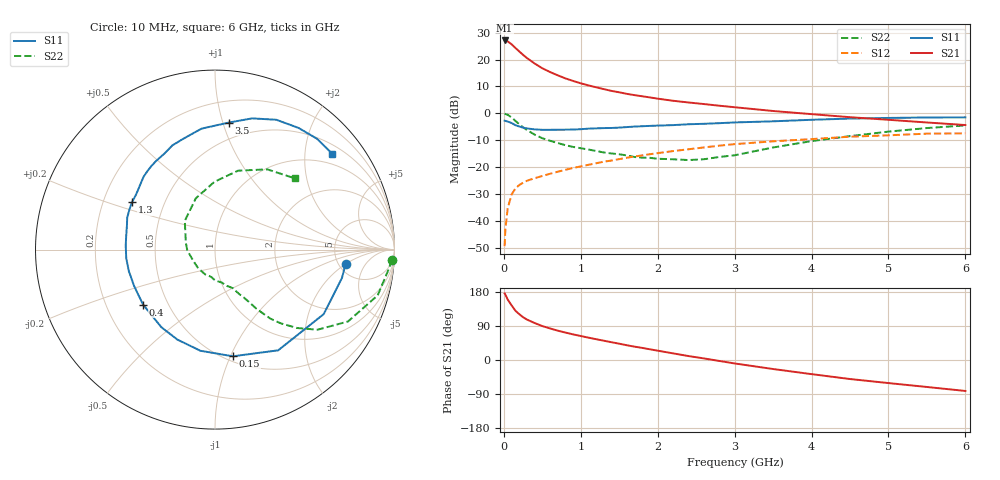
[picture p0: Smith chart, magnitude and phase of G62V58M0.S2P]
! SIEMENS Small Signal Semiconductors
! BFG193
! Si NPN RF Bipolar Junction Transistor in SOT223
! VCE = 2.5 V  IC = 8 mA
! Common Emitter S-Parameters:  August  1996
# GHz  S  MA  R  50
!  f  S11  S21  S12  S22
! GHz  MAG  ANG  MAG  ANG  MAG  ANG  MAG  ANG
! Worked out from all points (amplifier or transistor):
!   36 points, 10 MHz to 6 GHz, reference 50 ohm
!   highest |S21| = 27.1 dB at 10 MHz (marker M1)
!   |S21| within 3 dB of that: start of sweep to 158.8 MHz
!   unconditionally stable (mu >= 1): 940.8 MHz to 2.614 GHz
!   at 250 MHz: K = 0.47, MSG = 23.8 dB, |S12| = -25.8 dB
!   at 1.4 GHz: K = 1.08, MAG = 11.2 dB, |S12| = -17.5 dB
!   at 6 GHz: K = 0.89, MSG = 1.5 dB, |S12| = -7.4 dB
!   S11 on the Smith chart (normalised r, x): 10 MHz: 5.73, -2.01; 150 MHz: 0.55, -1.02; 400 MHz: 0.36, -0.30; 1.3 GHz: 0.32, +0.24; 3.5 GHz: 0.36, +1.05; 6 GHz: 0.71, +2.63
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0.01  0.7317 -6.4  22.67 175.7  0.0034 87.6  0.9864 -3.3
0.02  0.7249 -12.6  22.62 172.4  0.007 86.6  0.9741 -6.4
0.05  0.7043 -30.7  21.78 159.6  0.0171 76.8  0.9416 -15.7
0.1  0.6624 -57.9  19.29 144.4  0.0309 65.5  0.8422 -28.4
0.15  0.6027 -80.5  16.47 130.2  0.0401 56.1  0.725 -38.0
0.2  0.5695 -98.2  14.18 121.0  0.0465 52.3  0.6321 -43.7
0.25  0.5434 -112.7  12.23 112.9  0.0515 48.7  0.5499 -48.3
0.3  0.5256 -124.7  10.7 106.7  0.0558 47.2  0.4927 -51.3
0.4  0.5045 -142.6  8.456 97.6  0.0624 45.9  0.4023 -55.0
0.5  0.4943 -155.7  6.897 89.6  0.0685 45.2  0.3457 -57.1
0.6  0.4948 -165.9  5.871 83.3  0.0754 45.3  0.3094 -59.1
0.7  0.4968 -174.4  5.1 77.5  0.0823 45.7  0.2812 -61.5
0.9  0.5009 171.0  4.008 67.6  0.0966 46.1  0.2379 -65.1
1.1  0.5203 160.1  3.311 59.0  0.1106 45.4  0.2127 -71.9
1.3  0.5325 150.2  2.822 50.9  0.1265 44.0  0.1876 -78.3
1.7  0.5683 134.4  2.182 35.2  0.1578 39.7  0.1544 -97.4
2.2  0.6049 117.7  1.715 17.5  0.1991 31.5  0.1402 -131.4
2.8  0.6574 101.2  1.388 -2.5  0.251 20.2  0.1546 -178.8
3.5  0.7119 83.8  1.107 -23.8  0.3025 4.4  0.2323 136.4
4.5  0.8001 64.7  0.849 -50.2  0.3683 -15.5  0.3778 90.5
5.5  0.8392 47.4  0.677 -71.2  0.4199 -39.8  0.5336 56.9
6  0.844 39.3  0.607 -81.7  0.4258 -53.7  0.597 41.6
